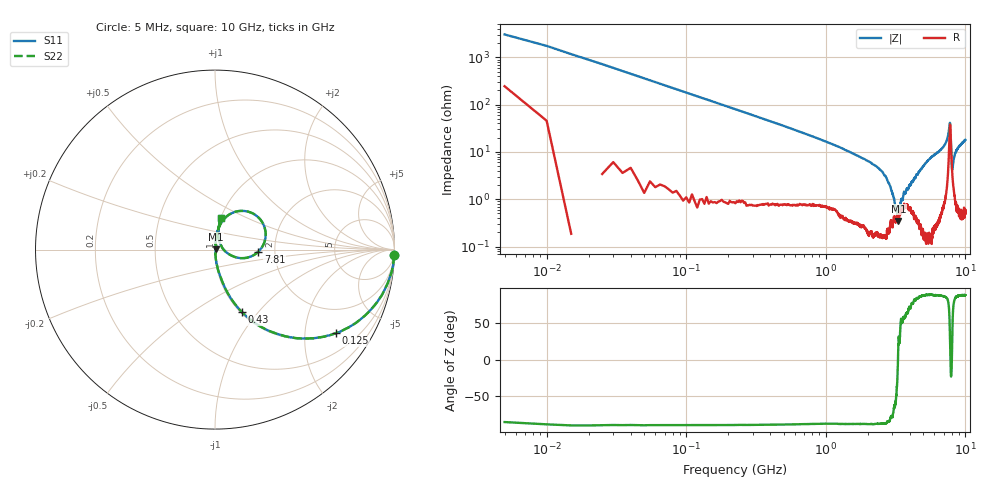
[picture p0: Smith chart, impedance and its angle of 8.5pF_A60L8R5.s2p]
! Amotech Co.,Ltd.
! http://www.amotech.co.kr/
! Part Number: A60L8R5
! These Parameters are Measured in Series Mode Connection
! Operation Temp=25[degC], DC Bias Voltage=0[V]
! Freq. Start=5[MHz] Stop=10[GHz], 2000[Steps]
! Date: Monday, July 14, 2020, 09:35:11
# GHZ S RI R 50.000000
!Freq.(Hz) S11(Real) S11(Imag) S21(Real) S21(Imag) S12(Real) S12(Imag) S22(Real) S22(Imag)
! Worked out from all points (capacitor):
!   2000 points, 5 MHz to 10 GHz, reference 50 ohm
!   read as one part in series: C = 8.82 pF near 55 MHz
!   lowest |Z| = 349 mohm at 3.315 GHz (marker M1)
!   series resonance near 3.29 GHz, so ESL is about 270 pH
!   S11 on the Smith chart (normalised r, x): 5 MHz: 6, -61; 125 MHz: 1.02, -2.89; 430 MHz: 1.02, -0.83; 7.81 GHz: 1.64, -0.04; 10 GHz: 1.01, +0.36
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0.005  0.9963 -0.0325  0.00368 0.0325  0.00368 0.0325  0.9963 -0.0325
0.07  0.8675 -0.3354  0.1325 0.3354  0.1325 0.3354  0.8675 -0.3354
0.125  0.6744 -0.4652  0.3256 0.4652  0.3256 0.4652  0.6744 -0.4652
0.26  0.3257 -0.4627  0.6743 0.4627  0.6743 0.4627  0.3257 -0.4627
0.43  0.1519 -0.3495  0.8481 0.3495  0.8481 0.3495  0.1519 -0.3495
1.675  0.01 -0.0829  0.99 0.0829  0.99 0.0829  0.01 -0.0829
2.685  0.0024 -0.0301  0.9976 0.0301  0.9976 0.0301  0.0024 -0.0301
2.92  0.00356 -0.0167  0.9964 0.0167  0.9964 0.0167  0.00356 -0.0167
3.315  0.00324 0.00127  0.9968 -0.00127  0.9968 -0.00127  0.00324 0.00127
3.34  0.00412 0.00208  0.9959 -0.00208  0.9959 -0.00208  0.00412 0.00208
3.465  0.00549 0.00789  0.9945 -0.00789  0.9945 -0.00789  0.00549 0.00789
3.64  0.00812 0.0119  0.9919 -0.0119  0.9919 -0.0119  0.00812 0.0119
5.005  0.00418 0.0504  0.9958 -0.0504  0.9958 -0.0504  0.00418 0.0504
6.67  0.0168 0.1096  0.9832 -0.1096  0.9832 -0.1096  0.0168 0.1096
7.32  0.0409 0.1581  0.9591 -0.1581  0.9591 -0.1581  0.0409 0.1581
7.64  0.1538 0.2157  0.8462 -0.2157  0.8462 -0.2157  0.1538 0.2157
7.735  0.2691 0.142  0.7309 -0.142  0.7309 -0.142  0.2691 0.142
7.81  0.2412 -0.0119  0.7588 0.0119  0.7588 0.0119  0.2412 -0.0119
8.035  0.0373 0.0156  0.9627 -0.0156  0.9627 -0.0156  0.0373 0.0156
8.335  0.018 0.0769  0.982 -0.0769  0.982 -0.0769  0.018 0.0769
8.78  0.0196 0.1148  0.9804 -0.1148  0.9804 -0.1148  0.0196 0.1148
10  0.0362 0.1734  0.9638 -0.1734  0.9638 -0.1734  0.0362 0.1734
